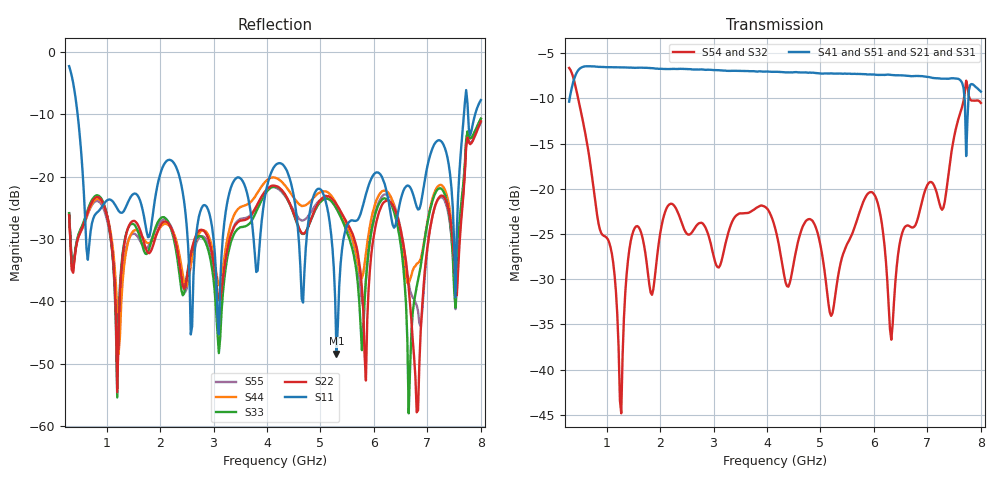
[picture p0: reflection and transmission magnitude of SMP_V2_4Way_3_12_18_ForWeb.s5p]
! Created Mon Mar 12 14:17:57 2018
# hz S ma R 50
! 5 Port Network Data from SP1.SP block
! freq  magS11  angS11  magS12  angS12  magS13  angS13  magS14  angS14
!  magS15  angS15
!  magS21  angS21  magS22  angS22  magS23  angS23
!  magS24  angS24  magS25  angS25
!  magS31  angS31  magS32  angS32
!  magS33  angS33  magS34  angS34  magS35  angS35
!  magS41  angS41
!  magS42  angS42  magS43  angS43  magS44  angS44  magS45  angS45
!  magS51  angS51  magS52  angS52  magS53  angS53  magS54  angS54
!  magS55  angS55
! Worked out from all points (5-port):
!   309 points, 300 MHz to 8 GHz, reference 50 ohm
!   strongest paths, dB at 300 MHz, 2.225 GHz, 4.15 GHz, 6.075 GHz, 8 GHz:
!     S41: -10.4, -6.7, -7.0, -7.4, -9.2
!     S51: -10.3, -6.7, -7.0, -7.4, -9.2
!     S21: -10.3, -6.7, -7.1, -7.4, -9.3
!     S31: -10.3, -6.7, -7.1, -7.5, -9.3
!     S54: -6.6, -21.7, -24.3, -21.7, -10.5
!     S32: -6.6, -21.7, -24.3, -21.7, -10.5
!   lowest |S11| = -48.4 dB at 5.3 GHz (marker M1), VSWR 1.01, Z = 50.3 - j0.237 ohm
!   |S11| at or under -10 dB: 458.4 MHz to 7.683 GHz (7.225 GHz wide, 177 % of centre); 7.76 GHz to 7.893 GHz (132.8 MHz wide, 1.7 % of centre)
